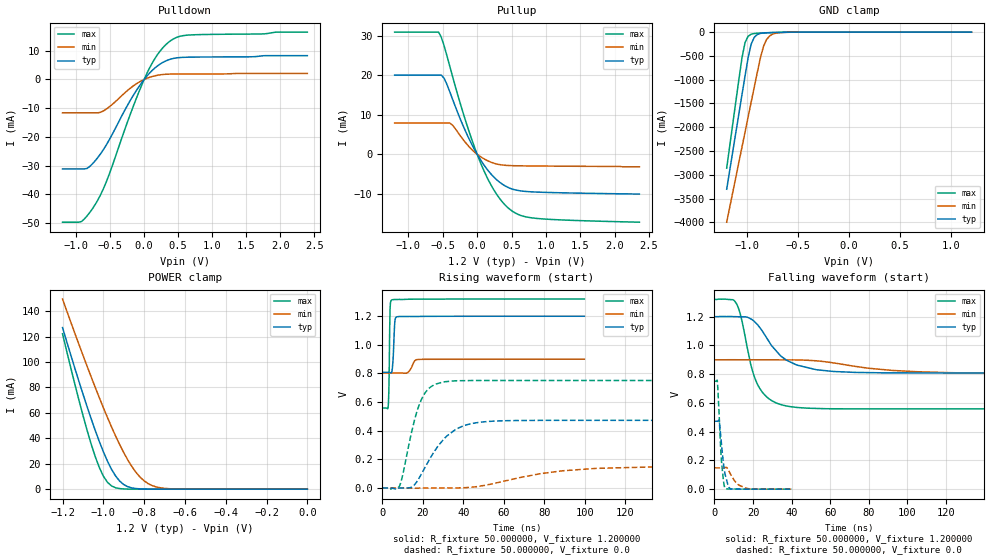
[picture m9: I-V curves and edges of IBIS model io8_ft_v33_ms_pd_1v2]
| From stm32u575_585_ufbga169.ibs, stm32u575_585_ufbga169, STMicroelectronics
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|   Model io8_ft_v33_ms_pd_1v2
[Model]  io8_ft_v33_ms_pd_1v2
Model_type I/O
Polarity   Non-Inverting
Enable   Active-Low
Vinl =   0.360000V
Vinh =   0.840000V
Vmeas =  0.600000V
Cref =   50.000000pF
Rref =   100.000000M
Vref =   0.0V
C_comp   2.887200pF   2.816900pF   2.935200pF
[Temperature Range]   25.000000   0.140000k   -40.000000
[Pullup Reference]   1.200000V   0.900000V   1.320000V
[Pulldown Reference]   0.0V   0.0V   0.0V
[POWER Clamp Reference]   1.200000V   0.900000V   1.320000V
[GND Clamp Reference]   0.0V   0.0V   0.0V
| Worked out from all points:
|   slope of the pulldown table from 0 to 0.18 V, typ, clamps not added: 40.7 ohm
|   slope of the pullup table from 0 to 0.18 V, typ, clamps not added: 39.5 ohm
|   GND clamp passes 1 mA (typ) near -0.51 V on its own axis
|   POWER clamp passes 1 mA (typ) near -0.86 V on its own axis
|   rising waveform, R_fixture 50.000000, V_fixture 1.200000: 20-80 % time 746ps typ, 2.06ns min, 445ps max; typ from 0.808 V to 1.2 V
|   rising waveform, R_fixture 50.000000, V_fixture 0.0: 20-80 % time 14.1ns typ, 33.7ns min, 7.83ns max; typ from 0 V to 0.472 V
|   falling waveform, R_fixture 50.000000, V_fixture 1.200000: 20-80 % time 15.4ns typ, 36.8ns min, 8.76ns max; typ from 1.2 V to 0.808 V
|   falling waveform, R_fixture 50.000000, V_fixture 0.0: 20-80 % time 2.49ns typ, 4.75ns min, 1.84ns max; typ from 0.472 V to 0 V
[Pulldown]
|Voltage   I(typ)   I(min)   I(max)
-1.2V     -31.16mA   -11.61mA   -49.71mA
-920mV    -31.16mA   -11.61mA   -49.48mA
-840mV    -31mA      -11.61mA   -47.54mA
-720mV    -28.33mA   -11.61mA   -43.58mA
-560mV    -22.95mA   -10.37mA   -35.89mA
-200mV    -7.146mA   -2.964mA   -11.89mA
0V        0A         0A         0A
160mV     4.047mA    1.298mA    7.361mA
360mV     6.87mA     1.87mA     13mA
480mV     7.543mA    1.91mA     14.69mA
640mV     7.765mA    1.923mA    15.46mA
2.4V      8.316mA    2.102mA    16.52mA
[Pullup]
|Voltage   I(typ)   I(min)   I(max)
-1.2V     20.06mA    7.936mA    30.97mA
-560mV    20.06mA    7.936mA    30.97mA
-480mV    19.26mA    7.936mA    27.49mA
-360mV    14.08mA    7.421mA    19.88mA
-160mV    5.494mA    2.768mA    8.045mA
40mV      -1.16mA    -508.1uA   -1.774mA
240mV     -5.73mA    -2.256mA   -8.953mA
360mV     -7.518mA   -2.715mA   -11.96mA
480mV     -8.639mA   -2.877mA   -14.04mA
640mV     -9.31mA    -2.942mA   -15.55mA
880mV     -9.601mA   -2.986mA   -16.29mA
2.36V     -10.1mA    -3.2mA     -17.23mA
[GND_clamp]
|Voltage   I(typ)   I(min)   I(max)
-1.2V     -3.305A    -3.998A    -2.862A
-1.05V    -1.316A    -2.418A    -539.3mA
-1.02V    -921mA     -2.103A    -218.8mA
-990mV    -539.5mA   -1.788A    -87.45mA
-960mV    -252.2mA   -1.474A    -44.37mA
-930mV    -110.5mA   -1.16A     -30.33mA
-870mV    -28.04mA   -549.1mA   -21.1mA
-840mV    -18.44mA   -305.6mA   -18.29mA
-810mV    -13.92mA   -159.7mA   -15.75mA
-780mV    -11.24mA   -82.36mA   -13.39mA
-600mV    -2.986mA   -4.279mA   -3.072mA
1.2V      30.28uA    18.17uA    37.27uA
[POWER_clamp]
|Voltage   I(typ)   I(min)   I(max)
-1.2V     127mA      149.4mA    122.2mA
-1.12V    84.97mA    114mA      70.27mA
-1.06V    55.51mA    88.42mA    35.67mA
-1.02V    37.63mA    72.04mA    17.17mA
-1V       29.51mA    64.13mA    10.3mA
-960mV    15.69mA    48.99mA    2.571mA
-900mV    3.624mA    28.77mA    182.8uA
-840mV    490.7uA    13.24mA    11.35uA
-800mV    116.8uA    6.532mA    1.77uA
-740mV    13.2uA     1.723mA    109.1nA
-620mV    167.3nA    79.35uA    0A
0V        0A         17.84nA    0A
[Ramp]
| variable   typ   min   max
dV/dt_r  0.28339/14.05621n   88.80588m/33.64508n 0.45045/7.82074n
dV/dt_f  0.23490/15.36475n   58.05600m/36.82443n 0.45672/8.74079n
R_load = 50.000000
[Rising Waveform]
R_fixture= 50.000000
V_fixture= 1.200000
V_fixture_min= 0.900000
V_fixture_max= 1.320000
|time   V(typ)   V(min)   V(max)
0s        808mV      802.7mV    558.2mV
2.803ns   808.1mV    802.7mV    557.9mV
3.203ns   808mV      802.7mV    675.7mV
3.804ns   806.5mV    802.7mV    1.252V
4.605ns   808mV      802.7mV    1.313V
5.205ns   881.8mV    802.7mV    1.315V
6.206ns   1.168V     802.7mV    1.316V
7.207ns   1.195V     802.7mV    1.316V
17.82ns   1.198V     897.5mV    1.319V
99.7ns    1.199V     899.4mV    1.319V
[Rising Waveform]
R_fixture= 50.000000
V_fixture= 0.0
V_fixture_min= 0.0
V_fixture_max= 0.0
|time   V(typ)   V(min)   V(max)
0s        2.199nV    207.3nV    1.402nV
8.408ns   -558.2uV   7.057uV    11.66mV
14.41ns   5.674mV    -1.065mV   388mV
19.22ns   95.87mV    -412.6uV   615.9mV
24.02ns   218.2mV    -105uV     707.3mV
30.63ns   345.2mV    63.76uV    741.6mV
40.24ns   434.8mV    1.692mV    749.5mV
57.66ns   468.4mV    39.75mV    750.6mV
105.7ns   472.3mV    136.8mV    750.7mV
299.1ns   472.4mV    148.1mV    750.8mV
[Falling Waveform]
R_fixture= 50.000000
V_fixture= 1.200000
V_fixture_min= 0.900000
V_fixture_max= 1.320000
|time   V(typ)   V(min)   V(max)
0s        1.199V     899.4mV    1.319V
10.81ns   1.199V     900mV      1.302V
13.21ns   1.199V     899.8mV    1.226V
18.62ns   1.186V     899.6mV    879mV
22.22ns   1.146V     899.6mV    731.9mV
28.23ns   1.027V     899.3mV    628.8mV
37.84ns   893.7mV    899mV      577.3mV
73.27ns   811.8mV    853.5mV    558.3mV
121.9ns   808mV      810mV      558.2mV
299.1ns   808mV      802.7mV    558.2mV
[Falling Waveform]
R_fixture= 50.000000
V_fixture= 0.0
V_fixture_min= 0.0
V_fixture_max= 0.0
|time   V(typ)   V(min)   V(max)
0s        472.4mV    148.1mV    750.8mV
1.522ns   472.1mV    148.1mV    748.9mV
2.482ns   472.2mV    148.1mV    502.3mV
3.524ns   331.5mV    148.1mV    217.5mV
4.725ns   173.6mV    147.9mV    54.57mV
5.365ns   114.1mV    149.1mV    9.344mV
8.248ns   2.53mV     106.5mV    1.034mV
11.93ns   552.1uV    35.31mV    725uV
17.54ns   259.7uV    3.402mV    271.1uV
39.88ns   2.199nV    207.3nV    1.402nV
